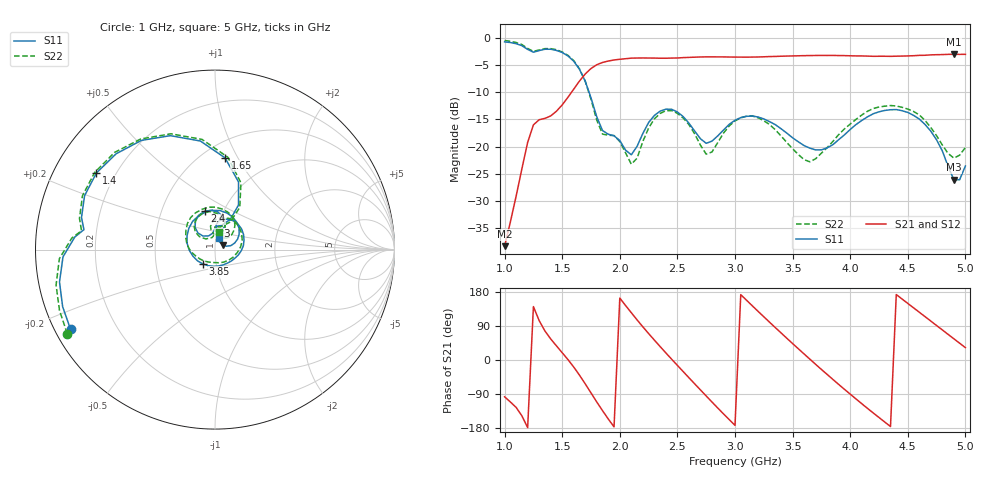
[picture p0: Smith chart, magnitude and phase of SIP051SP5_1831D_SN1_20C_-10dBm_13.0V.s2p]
# GHz  S  dB  R  50
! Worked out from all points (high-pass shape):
!   81 points, 1 GHz to 5 GHz, reference 50 ohm
!   highest |S21| = -3.01 dB at 4.9 GHz (marker M1); lowest = -38.3 dB at 1 GHz (marker M2)
!   |S21| within 3 dB of the highest: 1.731 GHz to end of sweep
!   lowest |S11| = -26.1 dB at 4.9 GHz (marker M3), VSWR 1.10, Z = 54.3 + j2.85 ohm
!   |S11| at or under -10 dB: 1.733 GHz to end of sweep
!   |S22| runs from -23.2 to -0.5 dB; largest |S21 - S12| = 0.0021
!   S11 on the Smith chart (normalised r, x): 1 GHz: 0.04, -0.26; 1.4 GHz: 0.13, +0.29; 1.65 GHz: 0.64, +0.89; 2.4 GHz: 0.82, +0.37; 3.85 GHz: 0.86, -0.14; 5 GHz: 1.03, +0.13
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1  -0.73 -151.1  -38.30 -97.1  -38.19 -97.4  -0.47 -150.4
1.25  -2.63 171.4  -15.99 140.9  -15.98 140.9  -2.48 172.0
1.4  -2.08 147.1  -14.35 55.6  -14.34 55.8  -1.98 147.3
1.65  -5.78 83.8  -7.93 -40.1  -7.94 -40.0  -5.68 82.1
1.7  -7.97 70.8  -6.63 -63.0  -6.63 -63.1  -7.99 68.7
1.8  -14.51 63.1  -4.94 -110.7  -4.94 -110.7  -15.12 61.1
2  -18.88 90.8  -3.93 163.4  -3.92 163.4  -19.06 87.5
2.15  -19.93 131.3  -3.70 105.8  -3.69 105.9  -22.12 130.7
2.35  -13.46 114.8  -3.74 35.4  -3.74 35.4  -13.89 120.3
2.4  -13.11 105.0  -3.74 18.7  -3.74 18.6  -13.39 109.3
2.55  -14.46 76.3  -3.63 -30.5  -3.63 -30.4  -14.74 77.0
2.7  -18.54 70.4  -3.51 -78.9  -3.51 -79.0  -19.73 67.6
3  -15.14 74.9  -3.53 -172.5  -3.52 -172.5  -15.27 86.3
3.35  -15.95 7.7  -3.41 85.6  -3.42 85.5  -16.89 5.8
3.55  -19.11 -35.2  -3.29 29.6  -3.28 29.5  -21.45 -55.9
3.7  -20.60 -77.5  -3.23 -11.5  -3.24 -11.5  -22.22 -116.1
3.85  -19.63 -130.3  -3.22 -51.3  -3.23 -51.4  -19.03 -160.5
4.05  -15.94 167.1  -3.31 -102.7  -3.31 -102.7  -14.99 156.7
4.35  -13.21 93.6  -3.39 -175.6  -3.40 -175.6  -12.44 98.9
4.65  -15.93 32.6  -3.19 114.4  -3.18 114.4  -15.19 50.3
4.9  -26.10 31.9  -3.01 55.9  -3.02 55.9  -22.11 58.1
5  -23.55 72.8  -3.02 32.7  -3.04 32.7  -20.15 76.7
